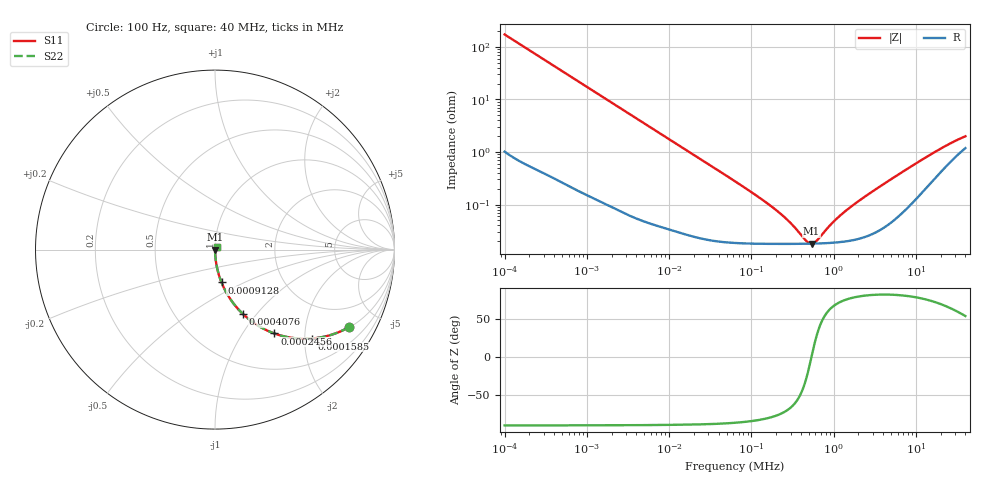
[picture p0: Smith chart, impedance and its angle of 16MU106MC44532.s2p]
!Components F PML CAP
!CONCATENATE F 0.1-40000kHz, at 20deg DC=0V
!Part Number F 16MU106MC44532
!Copyright(C) Rubycon Corporation. 20161129
# MHz S MA R 50
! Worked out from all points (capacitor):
!   561 points, 100 Hz to 40 MHz, reference 50 ohm
!   read as one part in series: C = 9.25 uF near 104.7 Hz
!   lowest |Z| = 18 mohm at 538.7 kHz (marker M1)
!   series resonance near 538.2 kHz, so ESL is about 9.5 nH
!   S11 on the Smith chart (normalised r, x): 100 Hz: 1.02, -3.44; 158.5 Hz: 1.01, -2.17; 245.6 Hz: 1.01, -1.40; 407.6 Hz: 1.01, -0.85; 912.8 Hz: 1.00, -0.38; 40 MHz: 1.02, +0.03
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0.0001  0.8624 -30.1  0.5012 59.6  0.5012 59.6  0.8624 -30.1
0.0001585162  0.7335 -42.5  0.6753 47.2  0.6753 47.2  0.7335 -42.5
0.000245552  0.5729 -54.7  0.8159 34.9  0.8159 34.9  0.5729 -54.7
0.0004075908  0.3892 -66.7  0.9183 22.9  0.9183 22.9  0.3892 -66.7
0.0005758105  0.2872 -72.9  0.9557 16.7  0.9557 16.7  0.2872 -72.9
0.0008716573  0.1948 -78.3  0.9792 11.2  0.9792 11.2  0.1948 -78.3
0.0009127527  0.1863 -78.8  0.9809 10.7  0.9809 10.7  0.1863 -78.8
0.002241283  0.07744 -85.0  0.9962 4.4  0.9962 4.4  0.07744 -85.0
0.007424854  0.0236 -87.7  0.9993 1.4  0.9993 1.4  0.0236 -87.7
0.06324555  0.00277 -86.0  0.9998 0.2  0.9998 0.2  0.00277 -86.0
0.204747  0.0007619 -76.4  0.9998 0.0  0.9998 0.0  0.0007619 -76.4
0.3028867  0.0004381 -66.0  0.9998 0.0  0.9998 0.0  0.0004381 -66.0
0.4691914  0.0002007 -26.6  0.9998 0.0  0.9998 0.0  0.0002007 -26.6
0.5387312  0.0001801 0.3  0.9998 -0.0  0.9998 -0.0  0.0001801 0.3
0.5512845  0.000181 5.0  0.9998 -0.0  0.9998 -0.0  0.000181 5.0
0.6185776  0.0002034 27.1  0.9998 -0.0  0.9998 -0.0  0.0002034 27.1
0.9363978  0.0004266 64.0  0.9998 -0.0  0.9998 -0.0  0.0004266 64.0
1.417512  0.0007663 74.9  0.9998 -0.0  0.9998 -0.0  0.0007663 74.9
2.246985  0.001317 79.7  0.9998 -0.1  0.9998 -0.1  0.001317 79.7
4.69589  0.002829 81.3  0.9996 -0.2  0.9996 -0.2  0.002829 81.3
17.45531  0.01017 70.8  0.9967 -0.6  0.9967 -0.6  0.01017 70.8
40  0.01968 52.6  0.9882 -0.9  0.9882 -0.9  0.01968 52.6
